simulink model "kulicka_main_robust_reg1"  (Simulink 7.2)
libraries: execlib x2

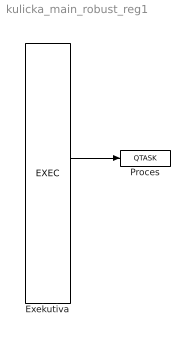
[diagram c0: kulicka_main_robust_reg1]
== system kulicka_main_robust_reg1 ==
  Exekutiva : execlib/EXEC  SystemSampleTime=-1  target=PC - Windows  tick=0.002  ntick0=10  ntick1=50  ntick2=100  ntick3=1200  pri0=5  pri1=9  pri2=13  pri3=18
  Proces : execlib/QTASK  SystemSampleTime=-1  factor=1  stack=2048  filename=kulicka_proces_robust_reg1  MDLOPEN=off
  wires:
  Exekutiva/4 -> Proces/1
